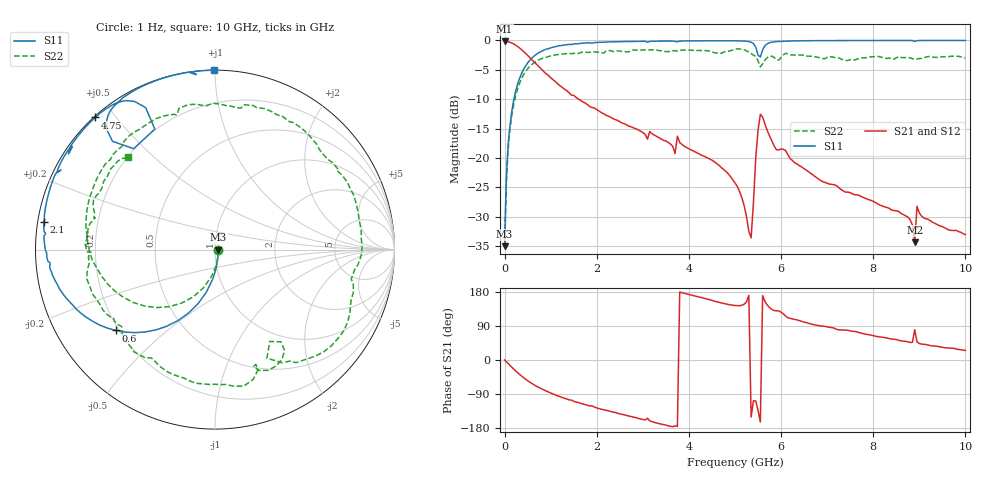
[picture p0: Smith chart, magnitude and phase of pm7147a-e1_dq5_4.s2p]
# GHz S DB R 50
! S-Parameters data
! Freq  dbS11  angS11  dbS21  angS21  dbS12  angS12  dbS22  angS22
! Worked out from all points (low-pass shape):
!   279 points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, 1 Hz to 10 GHz, reference 50 ohm
!   highest |S21| = -0.16 dB at 125.9 Hz (marker M1); lowest = -34.3 dB at 8.9 GHz (marker M2)
!   |S21| within 3 dB of the highest: start of sweep to 577.9 MHz
!   lowest |S11| = -35.0 dB at 125.9 Hz (marker M3), VSWR 1.04, Z = 51.8 - j1.23e-05 ohm
!   |S11| at or under -10 dB: start of sweep to 201.6 MHz
!   |S22| runs from -35.0 to -1.4 dB; largest |S21 - S12| = 6.3e-13
!   S11 on the Smith chart (normalised r, x): 1 Hz: 1.04, -0.00; 600 MHz: 0.19, -0.34; 2.1 GHz: 0.02, +0.08; 4.75 GHz: 0.00, +0.44; 10 GHz: 0.00, +0.99
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1e-09  -35.02 -0.0  -0.16 -0.0  -0.16 -0.0  -35.02 -0.0
1.259e-07  -35.02 -0.0  -0.16 -0.0  -0.16 -0.0  -35.02 -0.0
0.05011872  -21.50 -82.9  -0.19 -6.2  -0.19 -6.2  -22.17 -83.9
0.15  -12.37 -101.4  -0.42 -18.4  -0.42 -18.4  -13.08 -106.7
0.6  -2.94 -140.8  -3.33 -62.7  -3.33 -62.7  -4.05 -162.1
1.05  -1.16 -162.5  -6.68 -89.7  -6.68 -89.7  -2.55 163.3
1.7  -0.46 179.0  -10.47 -116.0  -10.47 -116.0  -2.00 126.9
2.1  -0.30 170.7  -12.30 -129.9  -12.30 -129.9  -2.08 106.8
3.35  -0.12 150.6  -16.58 -167.9  -16.58 -167.9  -1.72 48.4
4.75  -0.05 132.2  -21.94 149.5  -21.94 149.5  -2.00 -14.1
5.05  -0.07 127.9  -24.87 143.4  -24.87 143.4  -1.43 -32.2
5.35  -0.30 120.7  -33.60 -150.7  -33.60 -150.7  -2.21 -54.3
5.45  -1.11 116.0  -20.05 -108.1  -20.05 -108.1  -2.70 -59.4
5.55  -2.83 128.9  -12.58 -163.6  -12.58 -163.6  -4.50 -59.2
5.65  -0.90 132.0  -14.24 154.6  -14.24 154.6  -3.33 -55.4
6.1  -0.13 122.3  -18.76 116.0  -18.76 116.0  -2.19 -78.1
6.7  -0.04 115.6  -22.96 93.5  -22.96 93.5  -2.72 -110.8
8.35  -0.01 101.5  -28.60 56.3  -28.60 56.3  -3.01 -176.3
8.8  -0.01 98.0  -30.51 46.5  -30.51 46.5  -2.98 167.9
8.9  -0.17 96.1  -34.34 79.8  -34.34 79.8  -3.22 165.1
8.95  -0.04 97.9  -28.24 48.0  -28.24 48.0  -3.14 165.4
10  -0.00 90.4  -33.06 25.2  -33.06 25.2  -3.02 133.2
